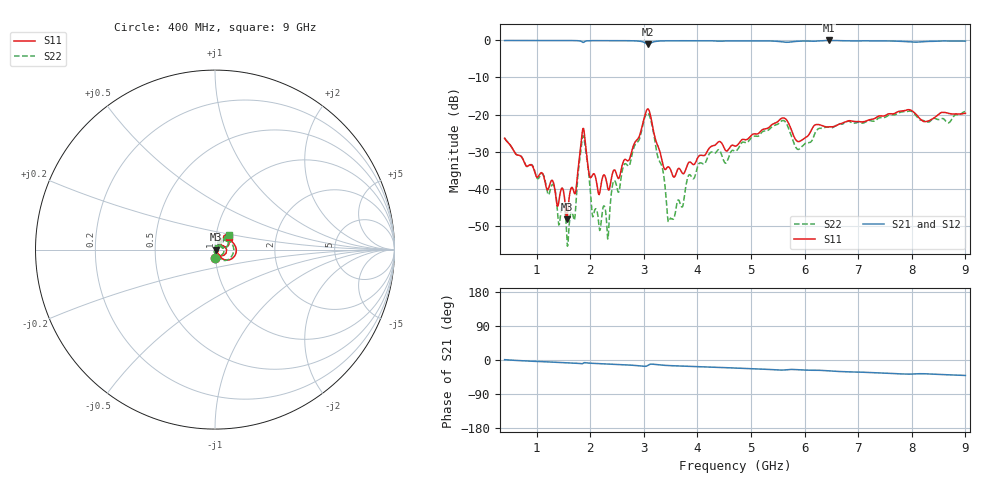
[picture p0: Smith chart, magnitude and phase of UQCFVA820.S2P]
!  Part Number  UQCFVA820  Mounting Orientation: Horizontal
!  Description: Ultra Low ESR Microwave capacitors
!  Application: Coupling, Bypass, Tuning, DC Block
!  Filters, Matching
# GHZ S DB R 50
! Freq  |S11|  S11 Ph  |S21|  S21 Ph  |S12|  S12 Ph  |S22|  S22 Ph
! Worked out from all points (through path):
!   801 points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, 400 MHz to 9 GHz, reference 50 ohm
!   highest |S21| = -0.01 dB at 6.452 GHz (marker M1); lowest = -1.0 dB at 3.077 GHz (marker M2)
!   group delay of S21, straight-line fit = 12.8 ps
!   lowest |S11| = -48.3 dB at 1.561 GHz (marker M3), VSWR 1.01, Z = 50.4 - j0.104 ohm
!   |S11| at or under -10 dB: start of sweep to end of sweep
!   |S22| runs from -55.5 to -19.0 dB; largest |S21 - S12| = 0.0098
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0.4  -26.39 -88.5  -0.03 0.9  -0.01 0.9  -26.34 -88.5
1.314  -38.47 -75.1  -0.03 -5.6  -0.01 -5.7  -39.00 -99.9
1.561  -48.30 -15.5  -0.03 -7.2  -0.01 -7.2  -52.76 -51.2
1.712  -41.39 17.5  -0.05 -8.1  -0.03 -8.2  -47.83 86.2
1.841  -26.00 25.6  -0.33 -10.1  -0.30 -10.1  -27.63 33.3
1.905  -27.39 -51.0  -0.24 -7.1  -0.22 -7.2  -28.89 -67.9
1.98  -36.28 -52.9  -0.08 -8.3  -0.06 -8.3  -37.43 -77.3
2.056  -35.99 -30.7  -0.06 -8.9  -0.04 -9.0  -47.37 -128.4
2.324  -39.80 0.7  -0.07 -10.6  -0.05 -10.7  -53.57 89.8
2.432  -35.12 27.5  -0.06 -11.3  -0.05 -11.4  -38.07 78.2
2.722  -32.26 51.5  -0.08 -13.2  -0.07 -13.3  -33.87 75.7
3.077  -18.49 -7.3  -1.05 -14.0  -1.03 -14.1  -19.65 -8.0
3.27  -28.84 -53.2  -0.18 -12.8  -0.16 -12.9  -32.00 -82.9
3.496  -34.83 -24.7  -0.11 -14.9  -0.09 -15.0  -47.94 -109.6
4.044  -31.00 38.2  -0.09 -18.1  -0.07 -18.3  -33.05 71.3
4.7  -28.51 46.8  -0.10 -21.2  -0.08 -21.4  -29.88 71.7
5.592  -20.91 35.9  -0.40 -26.5  -0.38 -26.7  -21.61 32.5
5.861  -27.20 27.9  -0.24 -25.6  -0.20 -25.6  -29.29 30.2
6.141  -23.77 61.3  -0.22 -27.1  -0.21 -27.4  -26.92 65.7
6.452  -23.32 49.1  -0.01 -28.7  -0.01 -28.9  -23.32 55.9
7.57  -19.79 53.6  -0.16 -35.1  -0.13 -35.4  -20.15 48.7
9  -19.65 42.1  -0.18 -40.8  -0.17 -41.3  -19.19 46.5
